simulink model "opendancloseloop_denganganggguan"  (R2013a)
settings: Solver=ode45  StartTime=0.0  StopTime=0.01  RelTol=1e-3
undefined symbols (not defined in the file): buckset4finalv2
libraries: powerlib x31, powerlib_meascontrol x3, fuzblock x1

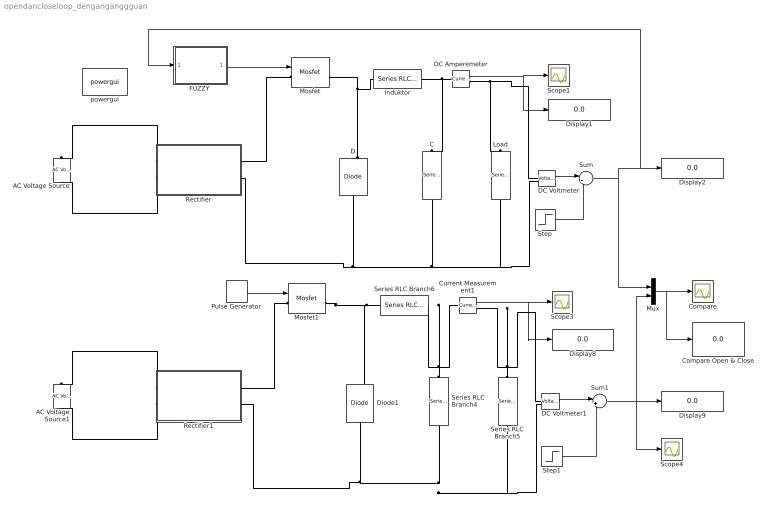
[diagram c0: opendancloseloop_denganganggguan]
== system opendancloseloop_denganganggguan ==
  AC Voltage Source : powerlib/Electrical Sources/AC Voltage Source  Amplitude=311.13  Phase=0  Frequency=50  SampleTime=0  Measurements=None
  AC Voltage Source1 : powerlib/Electrical Sources/AC Voltage Source  Amplitude=311.13  Phase=0  Frequency=50  SampleTime=0  Measurements=None
  C : powerlib/Elements/Series RLC Branch  LConnTagsString=__new0  RConnTagsString=__new0  BranchType=C  Resistance=1  Inductance=1e-3  SetiL0=off  InitialCurrent=0  Capacitance=1.35634e-05  Setx0=off  InitialVoltage=0  Measurements=None
  Compare : Scope
  Compare Open & Close : Display
  Current Measurement1 : powerlib/Measurements/Current Measurement  PhasorSimulation=off  OutputType=Complex  PSBequivalent=0
  D : powerlib/Power Electronics/Diode  Ron=0.001  Lon=0  Vf=0.8  IC=0  UseSnubber=off  Rs=500  Cs=250e-9  Measurements=on
  DC Amperemeter : powerlib/Measurements/Current Measurement  PhasorSimulation=off  OutputType=Complex  PSBequivalent=0
  DC Voltmeter : powerlib/Measurements/Voltage Measurement  PhasorSimulation=off  OutputType=Complex  PSBequivalent=0
  DC Voltmeter1 : powerlib/Measurements/Voltage Measurement  PhasorSimulation=off  OutputType=Complex  PSBequivalent=0
  Diode1 : powerlib/Power Electronics/Diode  Ron=0.001  Lon=0  Vf=0.8  IC=0  UseSnubber=off  Rs=500  Cs=250e-9  Measurements=on
  Display{1..2,8..9} (4 alike) : Display
  "FUZZY " : Subsystem
  Induktor : powerlib/Elements/Series RLC Branch  LConnTagsString=__new0  RConnTagsString=__new0  BranchType=L  Resistance=1  Inductance=0.0002304  SetiL0=off  InitialCurrent=0  Capacitance=1e-6  Setx0=off  InitialVoltage=0  Measurements=None
  Load : powerlib/Elements/Series RLC Branch  LConnTagsString=__new0  RConnTagsString=__new0  BranchType=R  Resistance=9  Inductance=1e-3  SetiL0=off  InitialCurrent=0  Capacitance=1e-6  Setx0=off  InitialVoltage=0  Measurements=None
  Mosfet : powerlib/Power Electronics/Mosfet  Ron=0.1  Lon=0  Rd=0.01  Vfd=0  IC=0  Rs=1e5  Cs=inf  Measurements=on
  Mosfet1 : powerlib/Power Electronics/Mosfet  Ron=0.1  Lon=0  Rd=0.01  Vfd=0  IC=0  Rs=1e5  Cs=inf  Measurements=on
  Mux : Mux  Inputs=2
  Pulse Generator : DiscretePulseGenerator  PulseType=Time based  Period=0.000025  PulseWidth=73
  Rectifier : Subsystem
  Rectifier1 : Subsystem
  Scope1 : Scope
  Scope3 : Scope
  Scope4 : Scope
  Series RLC Branch4 : powerlib/Elements/Series RLC Branch  LConnTagsString=__new0  RConnTagsString=__new0  BranchType=C  Resistance=1  Inductance=1e-3  SetiL0=off  InitialCurrent=0  Capacitance=1.35634e-05  Setx0=off  InitialVoltage=0  Measurements=None
  Series RLC Branch5 : powerlib/Elements/Series RLC Branch  LConnTagsString=__new0  RConnTagsString=__new0  BranchType=R  Resistance=9  Inductance=1e-3  SetiL0=off  InitialCurrent=0  Capacitance=1e-6  Setx0=off  InitialVoltage=0  Measurements=None
  Series RLC Branch6 : powerlib/Elements/Series RLC Branch  LConnTagsString=__new0  RConnTagsString=__new0  BranchType=L  Resistance=1  Inductance=0.0002304  SetiL0=off  InitialCurrent=0  Capacitance=1e-6  Setx0=off  InitialVoltage=0  Measurements=None
  Step : Step  Time=0.006  After=5  SampleTime=0
  Step1 : Step  Time=0.006  After=5  SampleTime=0
  Sum : Sum  Inputs=|++
  Sum1 : Sum  Inputs=|++
  powergui : powerlib/powergui  Priority=1  SimulationMode=Continuous  SolverType=Tustin  SampleTime=2.5e-5  frequency=60  SPID=off  DisableSnubberDevices=off  DisableRonSwitches=off  DisableVfSwitches=off  SwTol=0  Interpol=off  DisplayEquations=off  frequencyindice=0  Pbase=100e6  ErrMax=1e-4  Iterations=50  UnitsV=kV  UnitsW=MW  FunctionMessages=off  echomessages=off  HookPort=off  EnableUseOfTLC=off  x0status=blocks  RestoreLinks=warning  ResistiveCurrentMeasurement=off  Frange=[0:2:500]  Ylog=off  Xlog=on  ShowGrid=off  save=off  variable=ZData  ZoomFFT=off  StartTime=0.0  cycles=1  DisplayStyle=1  fundamental=60  FreqAxis=off  MaxFrequency=1000  frequencyindicesteady=1  RmsSteady=2  display=off  Ts=0  methode=off
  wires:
  DC Amperemeter/1 -> Scope1/1, Display1/1
  Current Measurement1/1 -> Scope3/1, Display8/1
  Pulse Generator/1 -> Mosfet1/1
  Mux/1 -> Compare Open & Close/1, Compare/1
  "FUZZY "/1(Out1) -> Mosfet/1
  Step/1 -> Sum/2
  DC Voltmeter/1 -> Sum/1
  DC Voltmeter1/1 -> Sum1/1
  Step1/1 -> Sum1/2
  Sum1/1 -> Mux/2, Scope4/1, Display9/1
  Sum/1 -> "FUZZY "/1(In1), Display2/1, Mux/1
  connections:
  Load/RConn1 -- DC Voltmeter/LConn2 -- C/RConn1 -- Rectifier/RConn2 -- D/LConn1
  D/RConn1 -- Induktor/LConn1 -- Mosfet/RConn1
  DC Amperemeter/RConn1 -- DC Voltmeter/LConn1 -- Load/LConn1
  DC Amperemeter/LConn1 -- Induktor/RConn1 -- C/LConn1
  Diode1/LConn1 -- Rectifier1/RConn2 -- Series RLC Branch4/RConn1 -- Series RLC Branch5/RConn1 -- DC Voltmeter1/LConn2
  Mosfet1/RConn1 -- Diode1/RConn1 -- Series RLC Branch6/LConn1
  Series RLC Branch5/LConn1 -- Current Measurement1/RConn1 -- DC Voltmeter1/LConn1
  Series RLC Branch4/LConn1 -- Current Measurement1/LConn1 -- Series RLC Branch6/RConn1
  Mosfet/LConn1 -- Rectifier/RConn1
  Rectifier/LConn1 -- AC Voltage Source/RConn1
  Rectifier/LConn2 -- AC Voltage Source/LConn1
  Rectifier1/LConn1 -- AC Voltage Source1/RConn1
  Rectifier1/LConn2 -- AC Voltage Source1/LConn1
  Mosfet1/LConn1 -- Rectifier1/RConn1

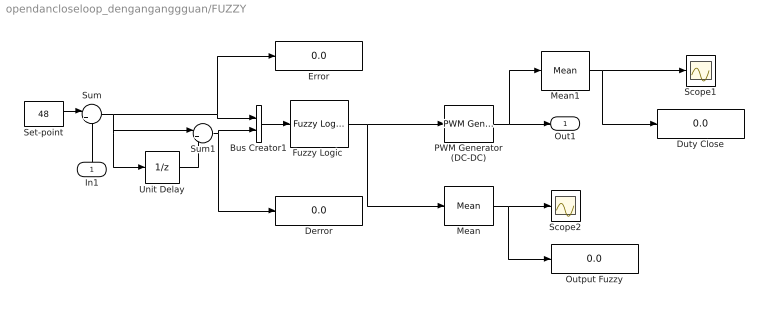
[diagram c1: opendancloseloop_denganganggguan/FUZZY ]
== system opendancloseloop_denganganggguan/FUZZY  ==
  In1 : Inport
  Bus Creator1 : BusCreator  Inputs=2
  Derror : Display
  Duty Close : Display
  Error : Display
  "Fuzzy Logic " : fuzblock/Fuzzy Logic  Controller  fis=[buckset4finalv2]
  Mean : powerlib_meascontrol/Measurements/Mean  Freq=40000  Vinit=0  Ts=0
  Mean1 : powerlib_meascontrol/Measurements/Mean  Freq=40000  Vinit=0  Ts=0
  Output Fuzzy : Display
  PWM Generator (DC-DC) : powerlib_meascontrol/Pulse & Signal Generators/PWM Generator (DC-DC)  Fsw=40000  Ts=0
  Scope1 : Scope
  Scope2 : Scope
  Set-point : Constant  Value=48
  Sum : Sum  Inputs=|+-
  Sum1 : Sum  Inputs=|+-
  Unit Delay : UnitDelay  SampleTime=-1
  Out1 : Outport
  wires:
  PWM Generator (DC-DC)/1 -> Out1/1, Mean1/1
  In1/1 -> Sum/2
  Unit Delay/1 -> Sum1/2
  Set-point/1 -> Sum/1
  Bus Creator1/1 -> "Fuzzy Logic "/1
  Sum/1 -> Error/1, Bus Creator1/1, Unit Delay/1, Sum1/1
  Sum1/1 -> Bus Creator1/2, Derror/1
  Mean/1 -> Scope2/1, Output Fuzzy/1
  Mean1/1 -> Duty Close/1, Scope1/1
  "Fuzzy Logic "/1 -> PWM Generator (DC-DC)/1, Mean/1

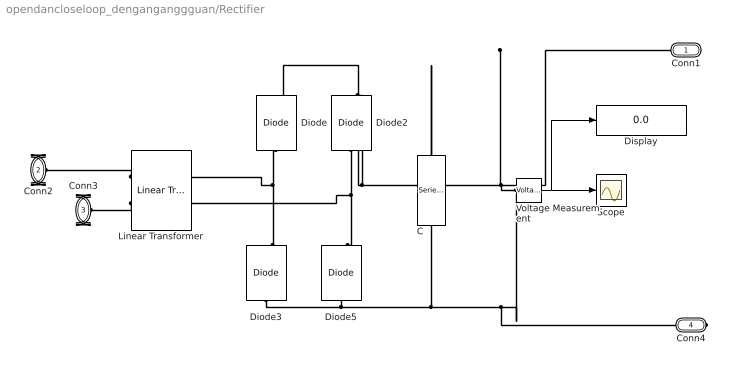
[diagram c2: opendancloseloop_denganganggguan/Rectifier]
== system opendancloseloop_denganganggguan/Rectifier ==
  C : powerlib/Elements/Series RLC Branch  LConnTagsString=__new0  RConnTagsString=__new0  BranchType=C  Resistance=1  Inductance=1e-3  SetiL0=off  InitialCurrent=0  Capacitance=4859e-5  Setx0=off  InitialVoltage=0  Measurements=None
  Diode{,2..3,5} (4 alike) : powerlib/Power Electronics/Diode  Ron=0.001  Lon=0  Vf=0.8  IC=0  UseSnubber=off  Rs=500  Cs=250e-9  Measurements=on
  Display : Display
  Linear Transformer : powerlib/Elements/Linear Transformer  LConnTagsString=a|b  RConnTagsString=A|B  UNITS=pu  NominalPower=[ 1000 50 ]  winding1="[ 220  0  0 ]"  winding2="[ 48  0  0 ]"  ThreeWindings=off  winding3=[ 315e3 0.002 0.08 ]  RmLm=[ 500 500 ]  Measurements=None  DataType=off
  Scope : Scope
  Voltage Measurement : powerlib/Measurements/Voltage Measurement  PhasorSimulation=off  OutputType=Complex  PSBequivalent=0
  Conn1 : PMIOPort  Port=1  Side=Right
  Conn2 : PMIOPort  Port=2  Side=Left
  Conn3 : PMIOPort  Port=3  Side=Left
  Conn4 : PMIOPort  Port=4  Side=Right
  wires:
  Voltage Measurement/1 -> Display/1, Scope/1
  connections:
  Linear Transformer/LConn1 -- Conn2/RConn1
  Linear Transformer/LConn2 -- Conn3/RConn1
  Voltage Measurement/LConn1 -- Conn1/RConn1 -- C/LConn1 -- Diode/RConn1 -- Diode2/RConn1
  Diode2/LConn1 -- Linear Transformer/RConn2 -- Diode5/RConn1
  Diode3/RConn1 -- Linear Transformer/RConn1 -- Diode/LConn1
  Diode3/LConn1 -- Diode5/LConn1 -- Conn4/RConn1 -- Voltage Measurement/LConn2 -- C/RConn1

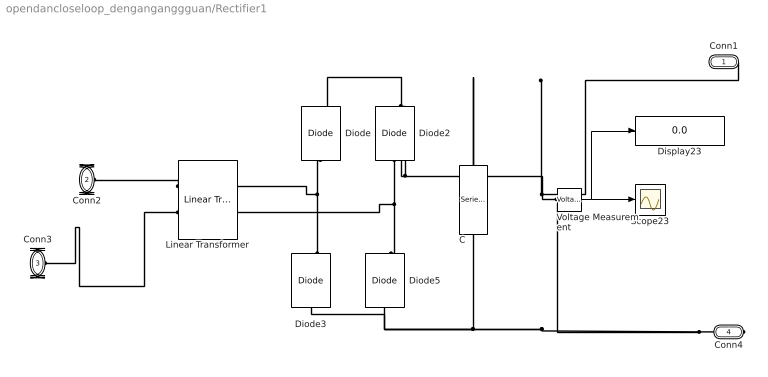
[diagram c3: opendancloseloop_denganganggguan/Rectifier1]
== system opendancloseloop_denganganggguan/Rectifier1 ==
  C : powerlib/Elements/Series RLC Branch  LConnTagsString=__new0  RConnTagsString=__new0  BranchType=C  Resistance=1  Inductance=1e-3  SetiL0=off  InitialCurrent=0  Capacitance=4859e-5  Setx0=off  InitialVoltage=0  Measurements=None
  Diode{,2..3,5} (4 alike) : powerlib/Power Electronics/Diode  Ron=0.001  Lon=0  Vf=0.8  IC=0  UseSnubber=off  Rs=500  Cs=250e-9  Measurements=on
  Display23 : Display
  Linear Transformer : powerlib/Elements/Linear Transformer  LConnTagsString=a|b  RConnTagsString=A|B  UNITS=pu  NominalPower=[ 1000 50 ]  winding1="[ 220  0  0 ]"  winding2="[ 48  0  0 ]"  ThreeWindings=off  winding3=[ 315e3 0.002 0.08 ]  RmLm=[ 500 500 ]  Measurements=None  DataType=off
  Scope23 : Scope
  Voltage Measurement : powerlib/Measurements/Voltage Measurement  PhasorSimulation=off  OutputType=Complex  PSBequivalent=0
  Conn1 : PMIOPort  Port=1  Side=Right
  Conn2 : PMIOPort  Port=2  Side=Left
  Conn3 : PMIOPort  Port=3  Side=Left
  Conn4 : PMIOPort  Port=4  Side=Right
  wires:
  Voltage Measurement/1 -> Display23/1, Scope23/1
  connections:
  Linear Transformer/LConn1 -- Conn2/RConn1
  Linear Transformer/LConn2 -- Conn3/RConn1
  Voltage Measurement/LConn1 -- C/LConn1 -- Diode/RConn1 -- Diode2/RConn1 -- Conn1/RConn1
  Diode2/LConn1 -- Diode5/RConn1 -- Linear Transformer/RConn2
  Diode3/RConn1 -- Linear Transformer/RConn1 -- Diode/LConn1
  Conn4/RConn1 -- Voltage Measurement/LConn2 -- Diode3/LConn1 -- Diode5/LConn1 -- C/RConn1
